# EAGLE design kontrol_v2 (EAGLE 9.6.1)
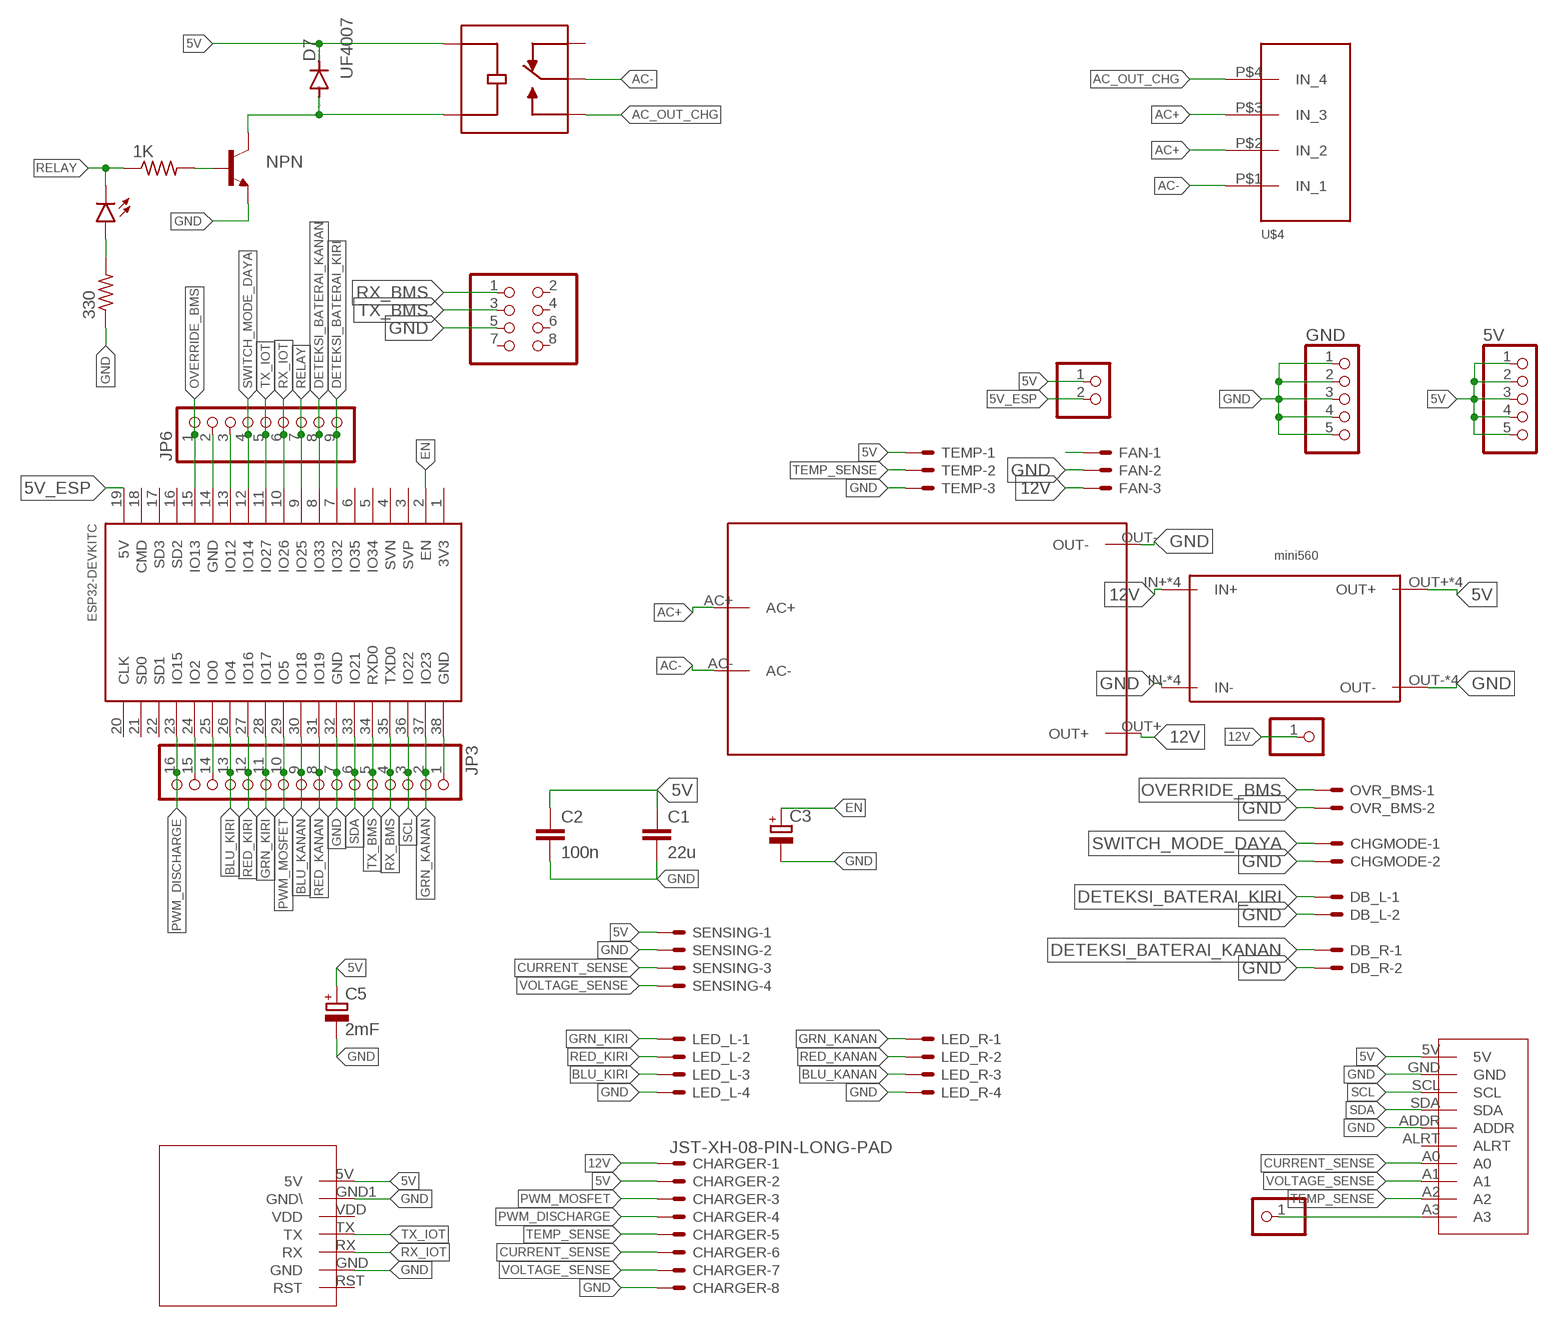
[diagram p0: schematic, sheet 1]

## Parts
1K  1k  R-US_0204/7  [0204/7]
5V  PINHD-1X5  [1X05]
330  6k  R-US_0204/7  [0204/7]
C1  22u  C2.5/5  [C2.5-5]
C2  100n  C2.5/6  [C2.5-6]
C3  CPOL-EUE2,5-6E  [E2,5-6E]
C5  2mF  CPOL-EUE3.5-10  [E3,5-10]
CHARGER  JST-XH-08-PIN-LONG-PAD  [JST-XH-08-PACKAGE-LONG-PAD]
CHGMODE  JST-XH-02-PIN-LONG-PAD  [JST-XH-02-PACKAGE-LONG-PAD]
D4  LED5MM  [LED_5MM]
D7  UF4007  BAS15  [DO34-7]
DB_L  JST-XH-02-PIN-LONG-PAD  [JST-XH-02-PACKAGE-LONG-PAD]
DB_R  JST-XH-02-PIN-LONG-PAD  [JST-XH-02-PACKAGE-LONG-PAD]
FAN  JST-XH-03-PIN-LONG-PAD  [JST-XH-03-PACKAGE-LONG-PAD]
GND  PINHD-1X5  [1X05]
HI_LINK1  HI_LINK  [HI_LINK]
JP2  PINHD-2X4  [2X04]
JP3  PINHD-1X16  [1X16]
JP4  PINHD-1X1  [1X01]
JP6  PINHD-1X9  [1X09]
JP7  PINHD-1X2  [1X02]
JP8  PINHD-1X1  [1X01]
K1  SRD-12VDC-SL-C  [RELAY_SRD-12VDC-SL-C]
LED_L  JST-XH-04-PIN-LONG-PAD  [JST-XH-04-PACKAGE-LONG-PAD]
LED_R  JST-XH-04-PIN-LONG-PAD  [JST-XH-04-PACKAGE-LONG-PAD]
MINI1  MINI560  [MINI560]
NPN  BC547A-NPN-TO92-CBE  [TO92-CBE]
OVR_BMS  JST-XH-02-PIN-LONG-PAD  [JST-XH-02-PACKAGE-LONG-PAD]
SENSING  JST-XH-04-PIN-LONG-PAD  [JST-XH-04-PACKAGE-LONG-PAD]
TEMP  JST-XH-03-PIN-LONG-PAD  [JST-XH-03-PACKAGE-LONG-PAD]
U$1  ESP32DEVKITC  [ESP32-DEVKITC]
U$2  ADS1115  [ADS1115]
U$3  SIM800V2  [SIM800V2]
U$4  TERMINAL_4P  [TERMINAL_4P]

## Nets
5V: 5V.1 5V.2 5V.3 5V.4 5V.5 C1.1 C2.1 C5.+ CHARGER.2 D7.C JP7.1 K1.COIL1 MINI1.OUT+ MINI1.OUT+1(OUT+) MINI1.OUT+2(OUT+) MINI1.OUT+3(OUT+) SENSING.1 TEMP.1 U$2.5V U$3.5V
5V_ESP: JP7.2 U$1.19(5V)
12V: CHARGER.1 FAN.3 HI_LINK1.OUT+ JP4.1 MINI1.IN+ MINI1.IN+1(IN+) MINI1.IN+2(IN+) MINI1.IN+3(IN+)
AC+: HI_LINK1.AC+ U$4.P$2(IN_2) U$4.P$3(IN_3)
AC-: HI_LINK1.AC- K1.COM U$4.P$1(IN_1)
AC_OUT_CHG: K1.NO U$4.P$4(IN_4)
BLU_KANAN: JP3.9 LED_R.3 U$1.30(IO18)
BLU_KIRI: JP3.13 LED_L.3 U$1.26(IO4)
CURRENT_SENSE: CHARGER.6 SENSING.3 U$2.A0
DETEKSI_BATERAI_KANAN: DB_R.1 JP6.8 U$1.8(IO33)
DETEKSI_BATERAI_KIRI: DB_L.1 JP6.9 U$1.7(IO32)
EN: C3.+ U$1.2(EN)
GND: 330.1 C1.2 C2.2 C3.- C5.- CHARGER.8 CHGMODE.2 DB_L.2 DB_R.2 FAN.2 GND.1 GND.2 GND.3 GND.4 GND.5 HI_LINK1.OUT- JP2.5 JP3.1 JP3.7 LED_L.4 LED_R.4 MINI1.IN- MINI1.IN-1(IN-) MINI1.IN-2(IN-) MINI1.IN-3(IN-) MINI1.OUT- MINI1.OUT-1(OUT-) MINI1.OUT-2(OUT-) MINI1.OUT-3(OUT-) NPN.E OVR_BMS.2 SENSING.2 TEMP.3 U$1.32(GND) U$1.38(GND) U$2.ADDR U$2.GND U$3.GND U$3.GND1(GND\)
GRN_KANAN: JP3.2 LED_R.1 U$1.37(IO23)
GRN_KIRI: JP3.11 LED_L.1 U$1.28(IO17)
N$1: 330.2 D4.A
N$2: FAN.1
N$8: JP6.2 U$1.14(GND)
N$9: JP6.3 U$1.13(IO12)
N$19: 1K.2 NPN.B
N$21: D7.A K1.COIL2 NPN.C
N$23: JP3.14 U$1.25(IO0)
N$24: JP3.15 U$1.24(IO2)
N$44: JP8.1 U$2.A3
OVERRIDE_BMS: JP6.1 OVR_BMS.1 U$1.15(IO13)
PWM_DISCHARGE: CHARGER.4 JP3.16 U$1.23(IO15)
PWM_MOSFET: CHARGER.3 JP3.10 U$1.29(IO5)
RED_KANAN: JP3.8 LED_R.2 U$1.31(IO19)
RED_KIRI: JP3.12 LED_L.2 U$1.27(IO16)
RELAY: 1K.1 D4.K(C) JP6.7 U$1.9(IO25)
RX_BMS: JP2.1 JP3.4 U$1.35(TXD0)
RX_IOT: JP6.6 U$1.10(IO26) U$3.RX
SCL: JP3.3 U$1.36(IO22) U$2.SCL
SDA: JP3.6 U$1.33(IO21) U$2.SDA
SWITCH_MODE_DAYA: CHGMODE.1 JP6.4 U$1.12(IO14)
TEMP_SENSE: CHARGER.5 TEMP.2 U$2.A2
TX_BMS: JP2.3 JP3.5 U$1.34(RXD0)
TX_IOT: JP6.5 U$1.11(IO27) U$3.TX
VOLTAGE_SENSE: CHARGER.7 SENSING.4 U$2.A1
Unconnected: JP2.2 JP2.4 JP2.6 JP2.7 JP2.8 K1.NC U$1.1(3V3) U$1.3(SVP) U$1.4(SVN) U$1.5(IO34) U$1.6(IO35) U$1.16(SD2) U$1.17(SD3) U$1.18(CMD) U$1.20(CLK) U$1.21(SD0) U$1.22(SD1) U$2.ALRT U$3.RST U$3.VDD

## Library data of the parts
1K 330 = rcl:R-US_: RESISTOR, American symbol; SPICEPREFIX: R
5V GND = pinhead:PINHD-1X5: PIN HEADER
C1 C2 = capacitor-wima:C: CAPACITOR
C3 C5 = rcl:CPOL-EU: POLARIZED CAPACITOR, European symbol; SPICEPREFIX: C
CHARGER = Rembrandt Electronics - JST XH Connectors v1-0:JST-XH-08-PIN: JST XH Connector 2 Pin Wire to board connector. Pitch: 2,54 mm, (0.100") Number of pins: 8 Created by Rembrandt Electronics www.rembrandtelectronics.com
CHGMODE DB_L DB_R OVR_BMS = JST XH Connectors v1-0:JST-XH-02-PIN: JST XH Connector 2 Pin
D4 = Sparkfun_LED:LED: LED (Generic)
D7 = diode:BAS15: DIODE
FAN TEMP = JST XH Connectors v1-0:JST-XH-03-PIN: JST XH Connector 2 Pin Wire to board connector. Pitch: 2,54 mm, (0.100") Number of pins: 3 Created by Rembrandt Electronics www.rembrandtelectronics.com
HI_LINK1 = Hi Link:HI_LINK
JP2 = pinhead:PINHD-2X4: PIN HEADER
JP3 = pinhead:PINHD-1X16: PIN HEADER
JP4 JP8 = pinhead:PINHD-1X1: PIN HEADER
JP6 = pinhead:PINHD-1X9: PIN HEADER
JP7 = pinhead:PINHD-1X2: PIN HEADER
K1 = TA_library:SRD-12VDC-SL-C: General Purpose Non Latching 12VDC SPDT Through Hole Relays RoHS Check availability; AVAILABILITY: Not in stock; DESCRIPTION: General Purpose Non Latching 12VDC SPDT Through Hole Relays RoHS; MF: Songle Relay; MP: SRD-12VDC-SL-C; PACKAGE: Package; PRICE: None
LED_L LED_R SENSING = JST XH Connectors v1-0:JST-XH-04-PIN: JST XH Connector 2 Pin Wire to board connector. Pitch: 2,54 mm, (0.100") Number of pins: 4 Created by Rembrandt Electronics www.rembrandtelectronics.com
MINI1 = mini560:MINI560
NPN = transistor:*-NPN-: NPN Transistror BF959 corrected 2008.03.06
U$1 = ESP32-DEVKITC:ESP32DEVKITC
U$2 = ADS1115:ADS1115
U$3 = sim800v2:SIM800V2
U$4 = TA_library:TERMINAL_4P

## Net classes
1 3A: width 3.302 mm, clearance 0.61 mm
3 HIGH Voltage: width 2.032 mm, clearance 2.54 mm
4 AC: width 2.032 mm, clearance 2.54 mm

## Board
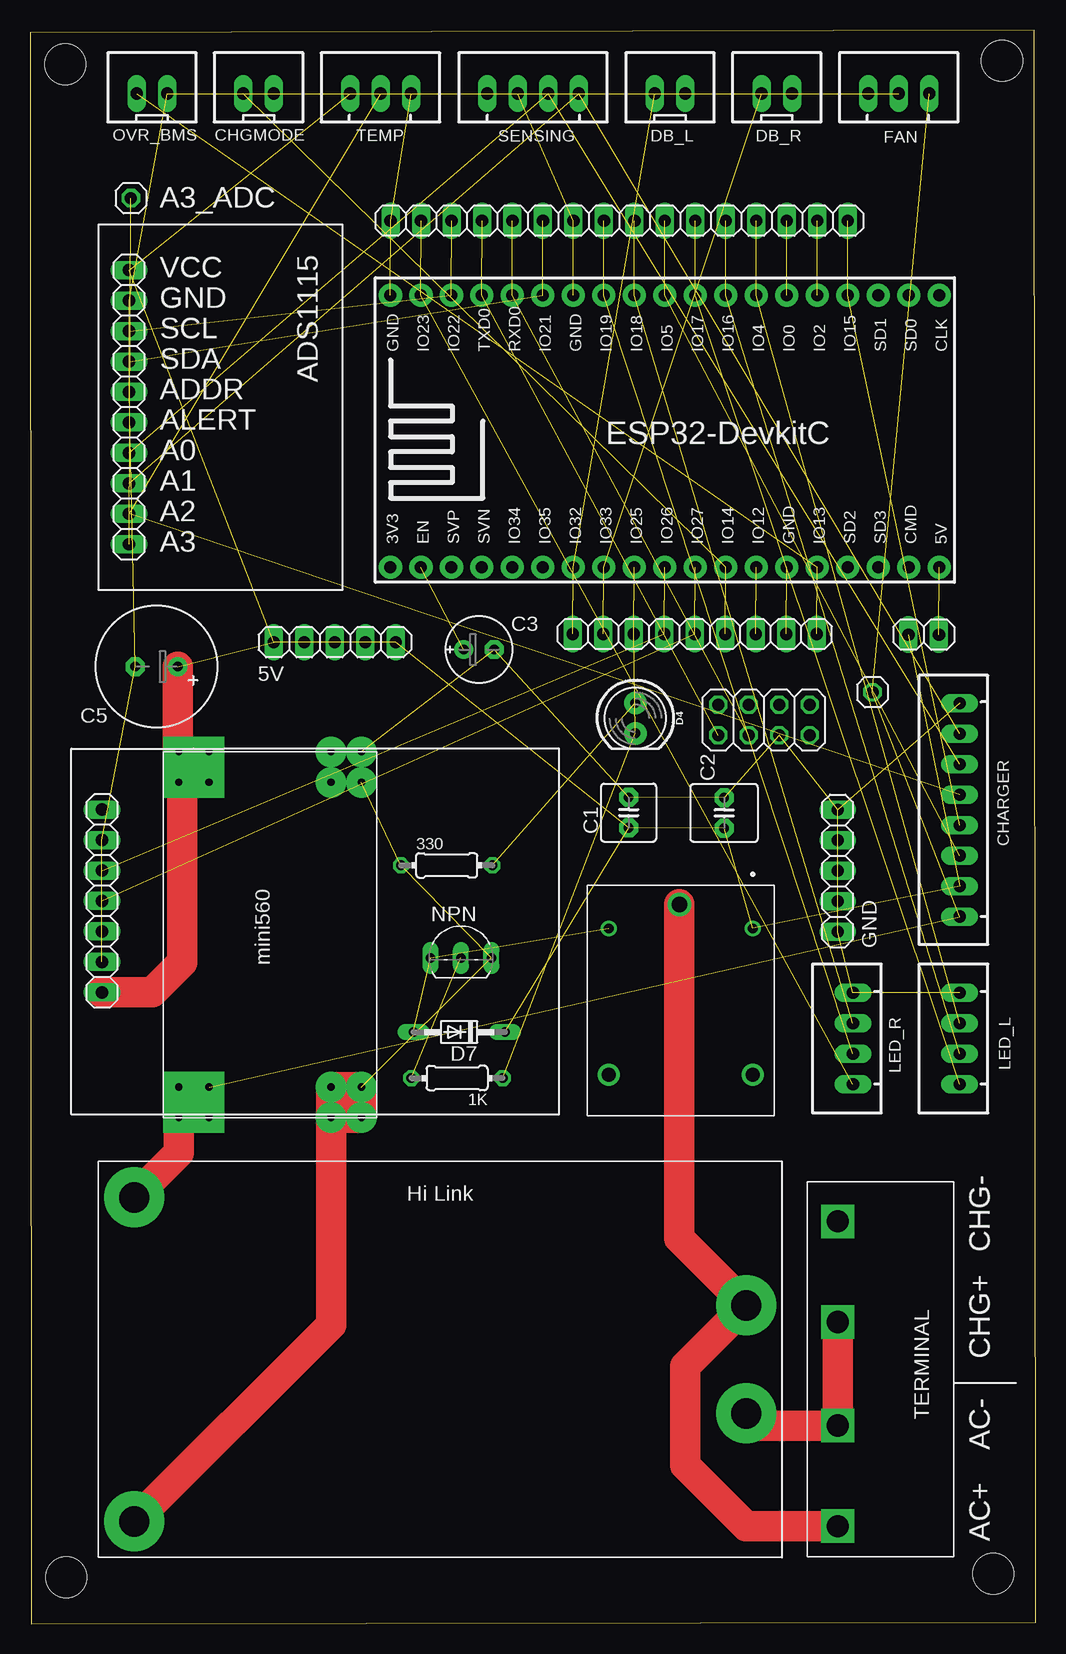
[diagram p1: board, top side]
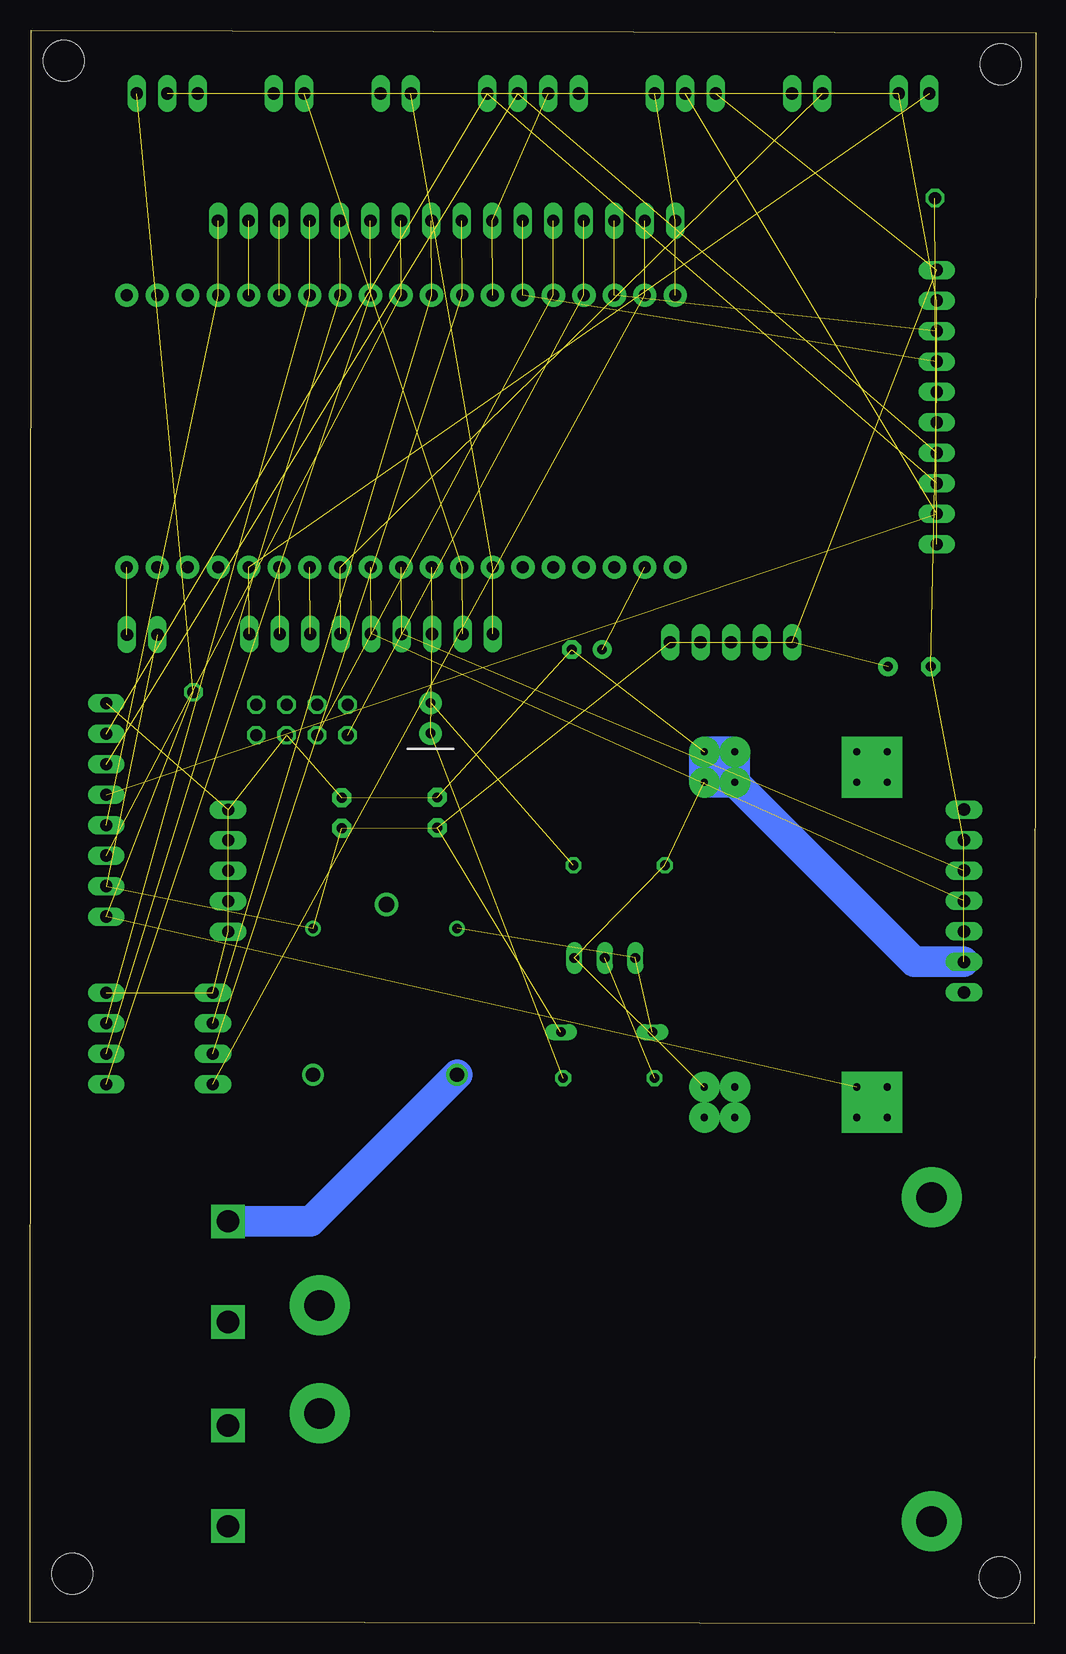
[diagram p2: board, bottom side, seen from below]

Size 83.82 x 132.8 mm. Coordinates in mm from the lower left corner, seen from the top.
Outline: 0.11,0 83.82,0.12 83.7,132.8 0,132.58 0.11,0
Copper layers (1*16): Top 0.035mm / dielectric 1.5mm / Bottom 0.035mm
Design rules "default *": minimum track width 12mil, minimum drill 0.35mm, track to track 12mil, track to pad 12mil, pad to pad 12mil, via to via 12mil, smd to smd 12mil, copper to edge 40mil, drill to drill 6mil, minimum pad ring 10mil, minimum via ring 8mil, stop-mask expansion 4mil, vias tented up to drill 0mil, thermal gap 10mil
Holes 3.4 mm at 3.02,3.85 2.92,129.94 81,130.21 80.29,4.15

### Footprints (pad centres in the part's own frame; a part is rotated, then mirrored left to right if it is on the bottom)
0204/7 = drill 0.813 octagon: 1 -3.81,0; 2 3.81,0
1X05 = drill 1.016 long: 1 -5.08,0; 2 -2.54,0; 3 0,0; 4 2.54,0; 5 5.08,0
C2.5-5 = drill 0.813 pad 1.6 octagon: 1 -1.27,0; 2 1.27,0
C2.5-6 = drill 0.813 pad 1.6 octagon: 1 -1.27,0; 2 1.27,0
E2,5-6E = drill 0.813 pad 1.575: + -1.27,0 | drill 0.813 pad 1.575 octagon: - 1.27,0
E3,5-10 = drill 0.813 pad 1.6: + -1.778,0 | drill 0.813 pad 1.6 octagon: - 1.778,0
JST-XH-08-PACKAGE-LONG-PAD = drill 1.016 long: 1 -8.89,0; 2 -6.35,0; 3 -3.81,0; 4 -1.27,0; 5 1.27,0; 6 3.81,0; 7 6.35,0; 8 8.89,0
JST-XH-02-PACKAGE-LONG-PAD = drill 1.016 long: 1 -1.27,0; 2 1.27,0
LED_5MM = drill 0.813 pad 1.88: A -1.27,0; K 1.27,0
DO34-7 = drill 0.813 long: A 3.81,0; C -3.81,0
JST-XH-03-PACKAGE-LONG-PAD = drill 1.016 long: 1 -2.54,0; 2 0,0; 3 2.54,0
HI_LINK = drill 2.54 pad 5: AC+ -23.67,4.49; AC- -23.67,-4.51; OUT+ 27.33,-13.51; OUT- 27.33,13.49
2X04 = drill 1.016 octagon: 1 -3.81,-1.27; 2 -3.81,1.27; 3 -1.27,-1.27; 4 -1.27,1.27; 5 1.27,-1.27; 6 1.27,1.27; 7 3.81,-1.27; 8 3.81,1.27
1X16 = drill 1.016 long: 1 -19.05,0; 2 -16.51,0; 3 -13.97,0; 4 -11.43,0; 5 -8.89,0; 6 -6.35,0; 7 -3.81,0; 8 -1.27,0; 9 1.27,0; 10 3.81,0; 11 6.35,0; 12 8.89,0; 13 11.43,0; 14 13.97,0; 15 16.51,0; 16 19.05,0
1X01 = drill 1.016 octagon: 1 0,0
1X09 = drill 1.016 long: 1 -10.16,0; 2 -7.62,0; 3 -5.08,0; 4 -2.54,0; 5 0,0; 6 2.54,0; 7 5.08,0; 8 7.62,0; 9 10.16,0
1X02 = drill 1.016 long: 1 -1.27,0; 2 1.27,0
RELAY_SRD-12VDC-SL-C = drill 0.8: COIL1 -6.1,6; COIL2 -6.1,-6 | drill 1.3: COM -8.1,-0.12 | drill 1.2: NC 6.1,6; NO 6.1,-6
JST-XH-04-PACKAGE-LONG-PAD = drill 1.016 long: 1 -3.81,0; 2 -1.27,0; 3 1.27,0; 4 3.81,0
MINI560 = drill 0.6 pad 2.54 square: IN+ 2.54,16.51; IN+1 2.54,13.97; IN+2 0,13.97; IN+3 0,16.51; OUT+ 27.94,16.51; OUT+1 27.94,13.97; OUT+2 30.48,16.51; OUT+3 30.48,13.97 | drill 0.6 pad 2.54: IN- 2.54,1.27; IN-1 0,3.81; IN-2 2.54,3.81; IN-3 0,1.27; OUT- 27.94,1.27; OUT-1 27.94,3.81; OUT-2 30.48,3.81; OUT-3 30.48,1.27
TO92-CBE = drill 0.813 long: B 0,0; C -2.54,0; E 2.54,0
ESP32-DEVKITC = drill 1 pad 1.93: 1 -22.87,-11.42; 2 -20.33,-11.42; 3 -17.79,-11.42; 4 -15.25,-11.42; 5 -12.71,-11.42; 6 -10.17,-11.42; 7 -7.63,-11.42; 8 -5.09,-11.42; 9 -2.55,-11.42; 10 -0.01,-11.42; 11 2.53,-11.42; 12 5.07,-11.42; 13 7.61,-11.42; 14 10.15,-11.42; 15 12.69,-11.42; 16 15.23,-11.42; 17 17.77,-11.42; 18 20.31,-11.42; 19 22.85,-11.42; 20 22.85,11.23; 21 20.31,11.23; 22 17.77,11.23; 23 15.23,11.23; 24 12.69,11.23; 25 10.15,11.23; 26 7.61,11.23; 27 5.07,11.23; 28 2.53,11.23; 29 -0.01,11.23; 30 -2.55,11.23; 31 -5.09,11.23; 32 -7.63,11.23; 33 -10.17,11.23; 34 -12.71,11.23; 35 -15.25,11.23; 36 -17.79,11.23; 37 -20.33,11.23; 38 -22.87,11.23
ADS1115 = drill 1.016 long: 5V -11.43,-7.62; A0 3.81,-7.62; A1 6.35,-7.62; A2 8.89,-7.62; A3 11.43,-7.62; ADDR -1.27,-7.62; ALRT 1.27,-7.62; GND -8.89,-7.62; SCL -6.35,-7.62; SDA -3.81,-7.62
SIM800V2 = drill 1.016 long: 5V 7.62,0; GND 5.08,0; GND1 -5.08,0; RST -7.62,0; RX -2.54,0; TX 0,0; VDD 2.54,0
TERMINAL_4P = drill 1.854 square: P$1 0,-3.81; P$2 0,4.572; P$3 0,13.208; P$4 0,21.59

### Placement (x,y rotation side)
1K  35.59,45.45 180 top
5V  25.4,81.78 0 top
330  34.72,63.18 0 top
C1  49.88,67.58 90 top
C2  57.84,67.55 90 top
C3  37.41,81.17 0 top
C5  10.54,79.74 180 top
CHARGER  77.47,67.81 90 top
CHGMODE  19.05,127.5 0 top
D4  50.44,75.45 270 top
D7  35.76,49.29 180 top
DB_L  53.34,127.5 0 top
DB_R  62.23,127.5 0 top
FAN  72.39,127.5 0 top
GND  67.31,62.73 90 top
HI_LINK1  36.02,22.01 180 top
JP2  61.16,75.3 0 top
JP3  49.1,116.9 0 top
JP4  70.21,77.61 0 top
JP6  55.4,82.46 180 top
JP7  74.47,82.41 0 top
JP8  8.41,118.78 0 top
K1  54.23,51.83 270 top
LED_L  77.47,48.76 90 top
LED_R  68.58,48.76 90 top
MINI1  28.89,42.16 90 top
NPN  35.92,55.46 0 top
OVR_BMS  10.16,127.5 0 top
SENSING  41.91,127.5 0 top
TEMP  29.21,127.5 0 top
U$1  52.91,99.46 0 top
U$2  15.88,101.36 270 top
U$3  5.99,60.21 270 top
U$4  67.31,11.93 0 top

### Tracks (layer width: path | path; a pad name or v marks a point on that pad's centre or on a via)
5V  (14 unrouted)
  Top 2.54: U$3.5V 10.19,52.59 12.7,55.11 12.7,69.79 MINI1.OUT+ | MINI1.OUT+2 MINI1.OUT+3 MINI1.OUT+1 MINI1.OUT+ | MINI1.OUT+2 MINI1.OUT+ | C5.+ 12.32,72.71 MINI1.OUT+2
5V_ESP  (1 unrouted)
12V  (3 unrouted)
  Top 2.54: HI_LINK1.OUT+ 12.38,39.22 MINI1.IN+3 | MINI1.IN+3 MINI1.IN+ MINI1.IN+1 MINI1.IN+2 MINI1.IN+3
AC+
  Top 2.54: HI_LINK1.AC+ 60.71,16.5 U$4.P$2 U$4.P$3
AC-
  Top 2.54: U$4.P$1 59.69,8.12 54.61,13.2 54.61,21.44 HI_LINK1.AC- 54.11,32.1 K1.COM
AC_OUT_CHG
  Bottom 2.54: K1.NO 60.44,33.52 U$4.P$4
BLU_KANAN  (2 unrouted)
BLU_KIRI  (2 unrouted)
CURRENT_SENSE  (2 unrouted)
DETEKSI_BATERAI_KANAN  (2 unrouted)
DETEKSI_BATERAI_KIRI  (2 unrouted)
EN  (1 unrouted)
GND  (30 unrouted)
  Top 2.54: HI_LINK1.OUT- 25.08,24.92 MINI1.IN-1 | MINI1.IN-1 MINI1.IN-2 MINI1.IN- MINI1.IN-3 MINI1.IN-1
  Bottom 2.54: U$3.GND 10.11,55.13 MINI1.OUT-1 | MINI1.OUT-1 MINI1.OUT- MINI1.OUT-3 MINI1.OUT-2 MINI1.OUT-1
GRN_KANAN  (2 unrouted)
GRN_KIRI  (2 unrouted)
N$1  (1 unrouted)
N$8  (1 unrouted)
N$9  (1 unrouted)
N$19  (1 unrouted)
N$21  (2 unrouted)
N$23  (1 unrouted)
N$24  (1 unrouted)
N$44  (1 unrouted)
OVERRIDE_BMS  (2 unrouted)
PWM_DISCHARGE  (2 unrouted)
PWM_MOSFET  (2 unrouted)
RED_KANAN  (2 unrouted)
RED_KIRI  (2 unrouted)
RELAY  (3 unrouted)
RX_BMS  (2 unrouted)
RX_IOT  (2 unrouted)
SCL  (2 unrouted)
SDA  (2 unrouted)
SWITCH_MODE_DAYA  (2 unrouted)
TEMP_SENSE  (2 unrouted)
TX_BMS  (2 unrouted)
TX_IOT  (2 unrouted)
VOLTAGE_SENSE  (2 unrouted)

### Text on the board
tNames: A3_ADC | CHG- | CHG+ | AC- | AC+

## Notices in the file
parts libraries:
Sparkfun_LED: Licensing: Creative Commons ShareAlike 4.0 International - https://creativecommons.org/licenses/by-sa/4.0
